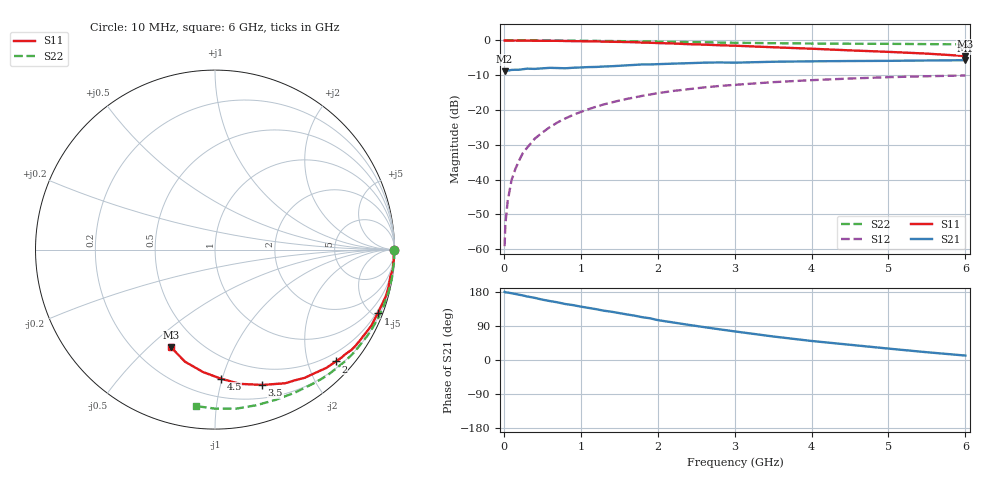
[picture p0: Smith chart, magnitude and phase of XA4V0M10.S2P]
! SIEMENS Discrete & RF Semiconductors
! BFY180
! Si NPN RF Bipolar Junction Transistor in MICRO-X
! VCE = 4 V  IC = 0.1 mA
! Common Emitter S-Parameters:  May  1997
# GHz  S  MA  R  50
!  f  S11  S21  S12  S22
! GHz  MAG  ANG  MAG  ANG  MAG  ANG  MAG  ANG
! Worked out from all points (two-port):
!   36 points, 10 MHz to 6 GHz, reference 50 ohm
!   highest |S21| = -5.68 dB at 6 GHz (marker M1); lowest = -8.9 dB at 10 MHz (marker M2)
!   |S21| within 3 dB of the highest: 17.64 MHz to 48.68 MHz (31.04 MHz wide, 93.6 % of centre); 50.74 MHz to end of sweep
!   lowest |S11| = -4.5 dB at 6 GHz (marker M3), VSWR 3.97, Z = 17.4 - j29.6 ohm
!   |S11| at or under -10 dB: nowhere
!   |S22| runs from -1.1 to 0.0 dB; largest |S21 - S12| = 0.4
!   S11 on the Smith chart (normalised r, x): 10 MHz: open; 1 GHz: 0.38, -5.27; 2 GHz: 0.32, -2.52; 3.5 GHz: 0.33, -1.36; 4.5 GHz: 0.33, -0.99; 6 GHz: 0.35, -0.59
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0.01  0.9968 -0.1  0.359 180.0  0.0011 89.0  0.999 -0.2
0.02  0.9997 -0.4  0.371 178.6  0.0023 91.3  0.9999 -0.4
0.05  0.9948 -1.0  0.368 178.0  0.0049 85.2  0.9996 -0.9
0.1  0.9964 -2.1  0.377 176.2  0.0098 87.9  0.9992 -1.9
0.15  0.9981 -3.5  0.379 174.3  0.0142 87.8  0.9999 -2.8
0.25  0.9969 -5.6  0.386 170.3  0.0243 85.8  0.9999 -4.8
0.4  0.9891 -8.4  0.39 164.1  0.0385 82.8  0.9983 -7.5
0.6  0.9885 -12.6  0.404 155.5  0.0569 78.3  0.9964 -11.3
0.8  0.9823 -17.0  0.398 147.7  0.0756 74.3  0.9934 -15.1
1  0.9743 -21.4  0.409 140.9  0.0937 70.2  0.9907 -18.9
1.1  0.9704 -23.4  0.414 137.5  0.1026 68.3  0.9876 -20.7
1.5  0.9533 -32.0  0.432 123.8  0.1366 60.1  0.978 -28.1
1.9  0.9268 -40.5  0.452 110.1  0.1668 52.6  0.9647 -35.3
2  0.9174 -42.8  0.456 105.3  0.1745 50.9  0.9623 -37.0
2.2  0.9047 -46.8  0.464 99.1  0.1878 46.9  0.9554 -40.6
2.8  0.8535 -58.6  0.483 81.1  0.2213 36.6  0.9338 -50.4
3.5  0.7985 -70.8  0.494 62.1  0.2513 25.9  0.9129 -60.8
4  0.7607 -79.5  0.501 50.2  0.2685 18.8  0.9028 -68.0
4.5  0.7198 -87.4  0.506 40.2  0.2835 12.2  0.8971 -75.2
5  0.6853 -95.6  0.509 30.1  0.2965 5.7  0.894 -82.4
5.5  0.6465 -105.0  0.515 20.5  0.3059 -0.9  0.8861 -89.9
6  0.5974 -114.1  0.52 11.7  0.3137 -7.5  0.8782 -97.1
